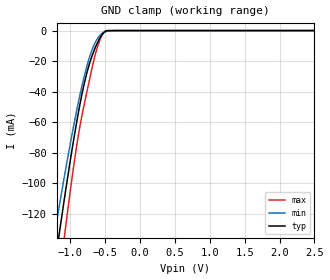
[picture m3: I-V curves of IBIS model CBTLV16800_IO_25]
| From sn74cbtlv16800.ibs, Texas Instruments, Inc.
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[Model]   CBTLV16800_IO_25
Model_type  Terminator
| variable   typ   min   max
C_comp   4.52pF   3.96pF   4.95pF
| C_tri-state   4.52pF   3.96pF   4.95pF
[Temperature Range]   40   100   -40
| Ambient temperature   25   85   -40
[Voltage range]   2.5   2.3   2.7
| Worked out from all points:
|   GND clamp passes 1 mA (typ) near -0.52 V on its own axis
[GND Clamp]
| CBTLV16800_IO_25
|   Voltage   I(typ)   I(min)   I(max)
-2.5V     -604.8mA   -520.6mA   -731.5mA
-1.245V   -160.1mA   -138.3mA   -195.7mA
-1.215V   -150.4mA   -130mA     -184mA
-1.16V    -132.9mA   -115mA     -162.7mA
-1.075V   -106.6mA   -92.51mA   -130.9mA
-915mV    -61.12mA   -53.38mA   -76.83mA
-775mV    -29.58mA   -25.07mA   -42.43mA
-700mV    -17.87mA   -13.84mA   -26.62mA
-620mV    -8.726mA   -5.827mA   -11.86mA
-560mV    -3.55mA    -2.332mA   -4.405mA
-500mV    -466.3uA   -767.1uA   -499.5uA
2.5V      1.214nA    60.76nA    11.78pA
